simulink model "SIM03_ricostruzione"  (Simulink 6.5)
settings: Solver=ode1  StartTime=0.0  StopTime=10  FixedStep=0.001  RelTol=1e-3
undefined symbols (not defined in the file or in its folder): poly

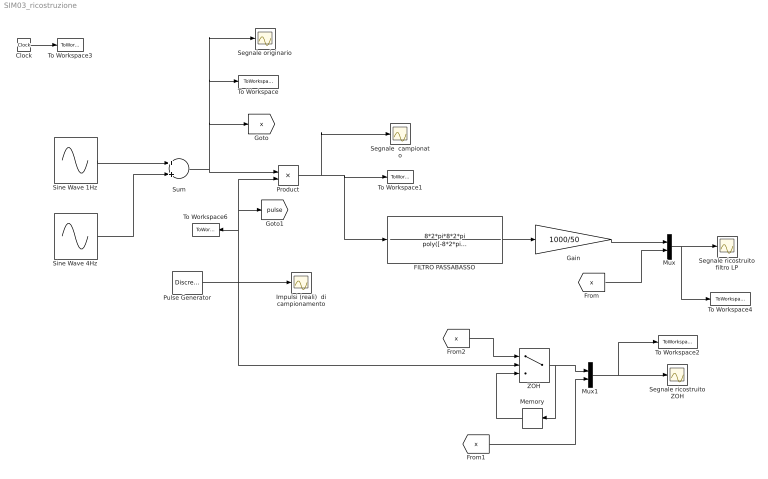
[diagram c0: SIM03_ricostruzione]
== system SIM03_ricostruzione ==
  Clock : Clock
  FILTRO PASSABASSO : TransferFcn  Numerator=8*2*pi*8*2*pi  Denominator=poly([-8*2*pi -8*2*pi ])
  Gain : Gain  Gain=1000/50
  Impulsi (reali)  di campionamento : Scope
  Memory : Memory  Orientation=left
  Mux : Mux  Inputs=2
  Mux1 : Mux  Inputs=2
  Product : Product
  Pulse Generator : DiscretePulseGenerator  PulseType=Time based  Period=0.02  PulseWidth=5  SampleTime=0.02
  Segnale  campionato : Scope
  Segnale originario : Scope
  Segnale ricostruito ZOH : Scope
  Segnale ricostruito filtro LP : Scope
  Sine Wave 1Hz : Sin  Frequency=2*pi  SampleTime=0
  Sine Wave 4Hz : Sin  Amplitude=0.5  Frequency=8*pi  SampleTime=0
  Sum : Sum
  To Workspace : ToWorkspace  VariableName=x  SampleTime=-1  SaveFormat=Array
  To Workspace1 : ToWorkspace  VariableName=xs  SampleTime=-1  SaveFormat=Array
  To Workspace2 : ToWorkspace  VariableName=xzoh  SampleTime=-1  SaveFormat=Array
  To Workspace3 : ToWorkspace  VariableName=tempo  SampleTime=-1  SaveFormat=Array
  To Workspace4 : ToWorkspace  VariableName=xlp  SampleTime=-1  SaveFormat=Array
  To Workspace6 : ToWorkspace  VariableName=samp  SampleTime=-1  SaveFormat=Array
  ZOH : Switch  Threshold=0.5
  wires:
  Sine Wave 1Hz/1 -> Sum/1
  Sine Wave 4Hz/1 -> Sum/2
  Sum/1 -> Product/1, To Workspace/1, Segnale originario/1, [x]
  Product/1 -> To Workspace1/1, FILTRO PASSABASSO/1, Segnale  campionato/1
  Pulse Generator/1 -> To Workspace6/1, Product/2, [pulse], Impulsi (reali)  di campionamento/1, ZOH/2
  Clock/1 -> To Workspace3/1
  [x] -> Mux/2
  Mux/1 -> Segnale ricostruito filtro LP/1, To Workspace4/1
  FILTRO PASSABASSO/1 -> Gain/1
  Gain/1 -> Mux/1
  Mux1/1 -> Segnale ricostruito ZOH/1, To Workspace2/1
  Memory/1 -> ZOH/3
  [x] -> ZOH/1
  ZOH/1 -> Memory/1, Mux1/1
  [x] -> Mux1/2
